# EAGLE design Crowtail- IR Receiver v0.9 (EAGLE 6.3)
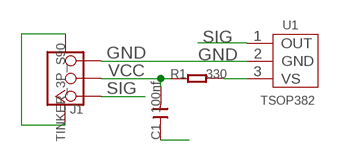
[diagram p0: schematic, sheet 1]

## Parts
C1  100nf  C-0603  [C0603]
J1  TINKER_3P_S90  [TINKER_3P_S90]
R1  330  R-0603  [0603]
U1  TSOP382  [3P-2.54-4.8X5X6.95H]

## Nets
GND: C1.1 J1.3 J1.SS1 J1.SS2 U1.2(GND)
N$1: R1.2 U1.3(VS)
SIG: J1.1 U1.1(OUT)
VCC: C1.2 J1.2 R1.1

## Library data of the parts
C1 = Discrete:C*: Ceramic Capacitors
J1 = Connector:TINKER_3P_S90
R1 = Discrete:R*
U1 = IC:TSOP382: IR Receiver Modules for Remote Control Systems

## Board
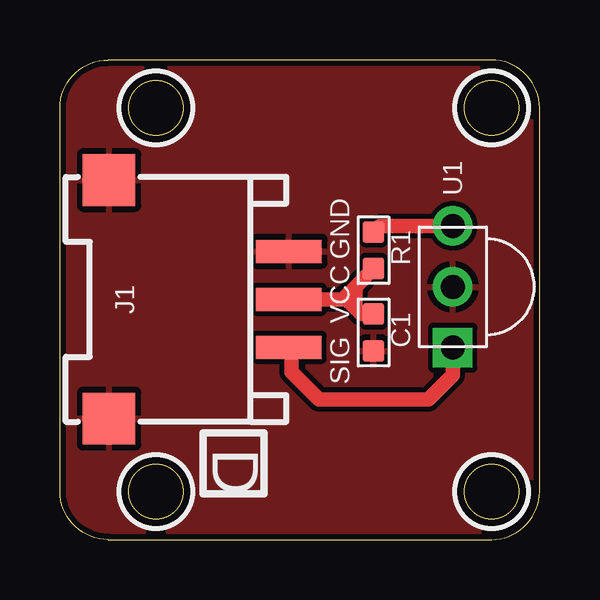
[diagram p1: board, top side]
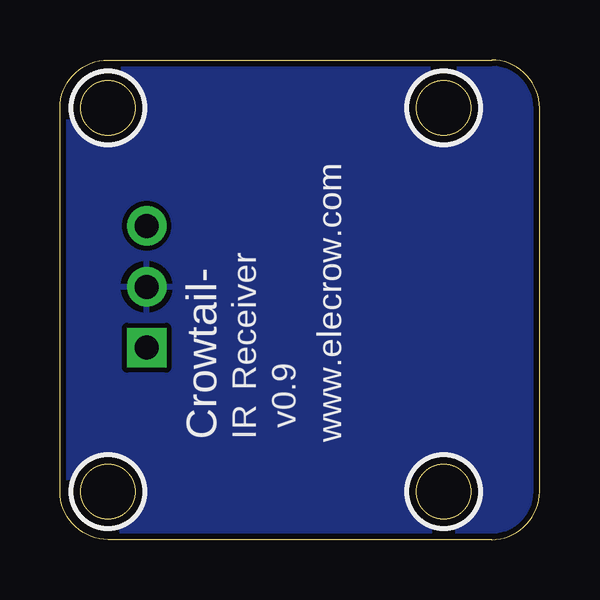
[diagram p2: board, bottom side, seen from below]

Size 20 x 20 mm. Coordinates in mm from the lower left corner, seen from the top.
Outline: 2,0 18,0 arc90 20,2 20,18 arc90 18,20 2,20 arc90 0,18 0,2 arc90 2,0
Outline: circle at 4,18 radius 1.14
Outline: circle at 4,2 radius 1.14
Outline: circle at 18,18 radius 1.14
Outline: circle at 18,2 radius 1.14
Copper layers (1*16): Top 0.035mm / dielectric 1.5mm / Bottom 0.035mm
Design rules "default *": minimum track width 10mil, minimum drill 10mil, track to track 8mil, track to pad 8mil, pad to pad 8mil, via to via 8mil, smd to smd 8mil, copper to edge 10mil, drill to drill 10mil, minimum pad ring 10mil, minimum via ring 8mil, stop-mask expansion 4mil, vias tented up to drill 0mil, thermal gap 10mil
tRestrict: area 2.5,16.5 to 5.5,19.5; area 2.5,0.5 to 5.5,3.5; area 16.5,16.5 to 19.5,19.5; area 16.5,0.5 to 19.5,3.5
bRestrict: area 2.5,16.5 to 5.5,19.5; area 2.5,0.5 to 5.5,3.5; area 16.5,16.5 to 19.5,19.5; area 16.5,0.5 to 19.5,3.5

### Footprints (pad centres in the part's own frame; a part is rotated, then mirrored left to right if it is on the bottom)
C0603 = smd 0.889 x 0.889: 1 -0.762,0; 2 0.762,0
TINKER_3P_S90 = smd 0.965 x 2.74: 1 -1.984,-4.545; 2 0.016,-4.545; 3 2.016,-4.545 | smd 2.159 x 2.184: SS1 -4.958,2.955; SS2 4.99,2.955
0603 = smd 0.889 x 0.889: 1 -0.762,0; 2 0.762,0
3P-2.54-4.8X5X6.95H = drill 1 pad 1.65 square: 1 -2.54,0 | drill 1 pad 1.65: 2 0,0; 3 2.54,0

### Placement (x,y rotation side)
C1  13.08,8.64 90 top
J1  5,10 90 top
R1  13.08,12.06 90 top
U1  16.38,10.54 90 top

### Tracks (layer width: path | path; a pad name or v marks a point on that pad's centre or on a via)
GND
  pour Top: 0,0 20.32,0 20.32,20.32 0,20.32
  pour Bottom: 0,0 20.32,0 20.32,20.32 0,20.32
N$1
  Top 0.61: U1.3 13.34,13.08 R1.2
SIG
  Top 0.61: U1.1 16.38,6.86 15.37,5.84 10.79,5.84 9.65,6.99 9.65,7.91 J1.1
VCC
  Top 0.61: J1.2 11.79,10.02 11.87,10.1 | 11.87,10.1 12.32,10.54 | 12.32,10.54 R1.1 | C1.2 12.57,9.4 12.32,9.65 | 12.32,9.65 11.87,10.1 | 12.32,10.54 12.32,9.65

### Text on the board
tPlace: GND | VCC | SIG | D
bPlace: v0.9 | Receiver | www.elecrow.com | IR | Crowtail-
